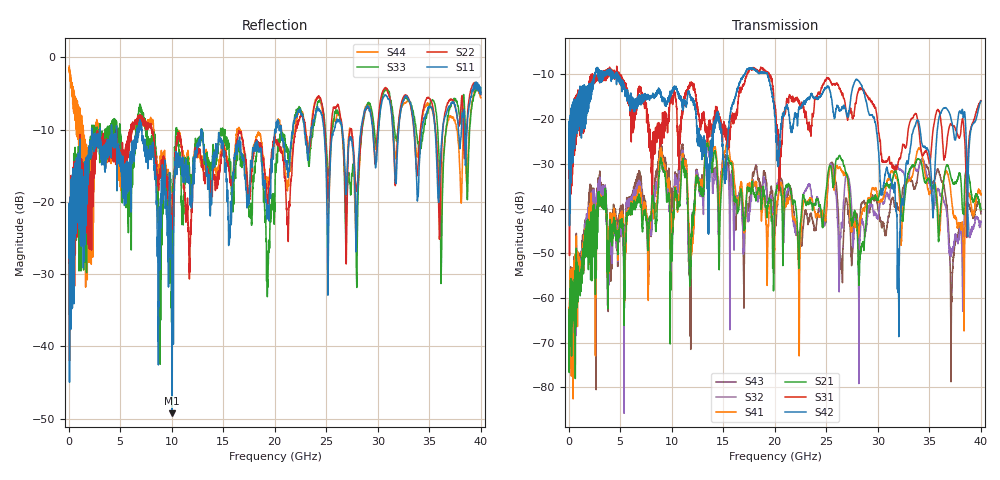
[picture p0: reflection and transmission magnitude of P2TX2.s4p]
!Agilent Technologies,N5245A,MY49151084,A.09.20.08
!Agilent N5245A: A.09.20.08
!Date: Thursday, March 01, 2012 13:21:25
!Correction: S11(Full 4 Port(1,2,3,4))
!S12(Full 4 Port(1,2,3,4))
!S13(Full 4 Port(1,2,3,4))
!S14(Full 4 Port(1,2,3,4))
!S21(Full 4 Port(1,2,3,4))
!S22(Full 4 Port(1,2,3,4))
!S23(Full 4 Port(1,2,3,4))
!S24(Full 4 Port(1,2,3,4))
!S31(Full 4 Port(1,2,3,4))
!S32(Full 4 Port(1,2,3,4))
!S33(Full 4 Port(1,2,3,4))
!S34(Full 4 Port(1,2,3,4))
!S41(Full 4 Port(1,2,3,4))
!S42(Full 4 Port(1,2,3,4))
!S43(Full 4 Port(1,2,3,4))
!S44(Full 4 Port(1,2,3,4))
!S4P File: Measurements: <S11,S12,S13,S14>,
!<S21,S22,S23,S24>,
!<S31,S32,S33,S34>,
!<S41,S42,S43,S44>:
# Hz S  dB  R 50
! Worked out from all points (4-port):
!   3996 points, 50 MHz to 40 GHz, reference 50 ohm
!   strongest paths, dB at 50 MHz, 10.04 GHz, 20.03 GHz, 30.02 GHz, 40 GHz:
!     S42: -25.2, -13.6, -19.4, -25.7, -16.0
!     S31: -24.5, -15.1, -16.9, -21.3, -15.9
!     S21: -62.5, -51.8, -37.8, -37.9, -40.3
!     S41: -64.5, -44.1, -42.1, -38.0, -37.0
!     S32: -69.2, -49.8, -39.7, -41.9, -42.9
!     S43: -65.8, -41.3, -43.1, -40.2, -41.2
!   lowest |S11| = -49.3 dB at 10.05 GHz (marker M1), VSWR 1.01, Z = 49.7 + j0.172 ohm
!   |S11| at or under -10 dB: start of sweep to 2.239 GHz; 7.093 GHz to 12.85 GHz (5.756 GHz wide, 57.7 % of centre); 12.85 GHz to 20.01 GHz (7.155 GHz wide, 43.6 % of centre)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
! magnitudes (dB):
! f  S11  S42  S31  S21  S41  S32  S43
! 50 MHz  -21.5  -25.2  -24.5  -62.5  -64.5  -69.2  -65.8
! 2.99 GHz  -12.1  -9.7  -10.8  -37.0  -36.6  -33.9  -33.9
! 10.05 GHz  -49.3  -14.1  -16.0  -51.3  -44.3  -45.1  -37.2
! 28.06 GHz  -16.7  -11.3  -14.1  -48.3  -46.0  -46.2  -43.3
! 32.02 GHz  -10.2  -59.5  -29.3  -34.3  -35.5  -31.1  -40.2
! 33.71 GHz  -15.1  -20.8  -18.8  -29.7  -28.3  -31.5  -34.8
! 40 GHz  -5.1  -16.0  -15.9  -40.3  -37.0  -42.9  -41.2
